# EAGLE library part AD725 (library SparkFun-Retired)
RGB component to NTSC/PAL Encoder Not in catalog
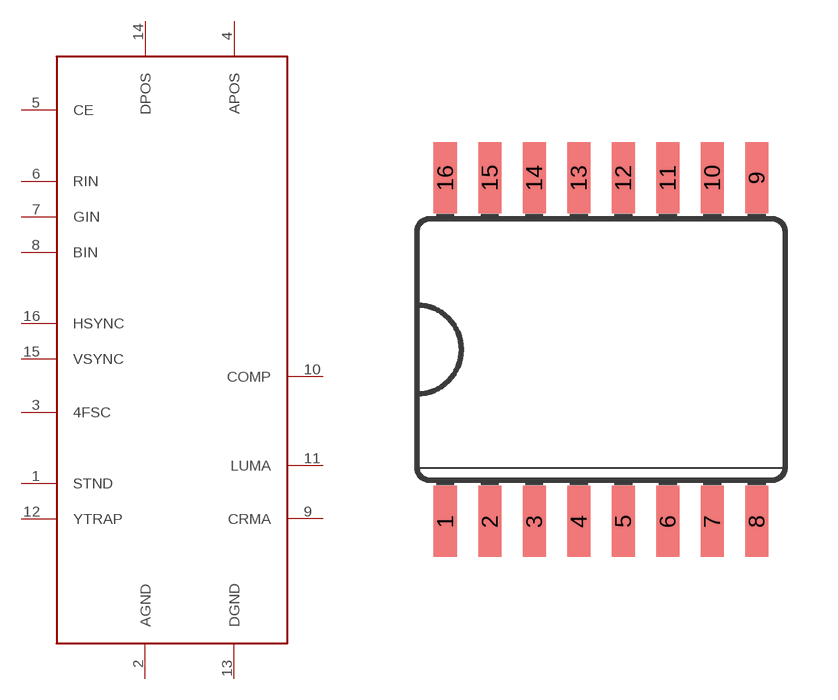
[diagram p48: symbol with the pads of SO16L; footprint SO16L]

Designator prefix -

## AD725  [SO16L]
1  STND
2  AGND
3  4FSC
4  APOS
5  CE
6  RIN
7  GIN
8  BIN
9  CRMA
10  COMP
11  LUMA
12  YTRAP
13  DGND
14  DPOS
15  VSYNC
16  HSYNC

## Footprint SO16L (pad centres in mm)
Small Outline Package .300 SIOC Source: http://www.maxim-ic.com/cgi-bin/packages?pkg=16%2FSOIC%2E300&Type=Max
smd 0.66 x 2.032: 1 -4.445,-4.902; 2 -3.175,-4.902; 3 -1.905,-4.902; 4 -0.635,-4.902; 5 0.635,-4.902; 6 1.905,-4.902; 7 3.175,-4.902; 8 4.445,-4.902; 9 4.445,4.902; 10 3.175,4.902; 11 1.905,4.902; 12 0.635,4.902; 13 -0.635,4.902; 14 -1.905,4.902; 15 -3.175,4.902; 16 -4.445,4.902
